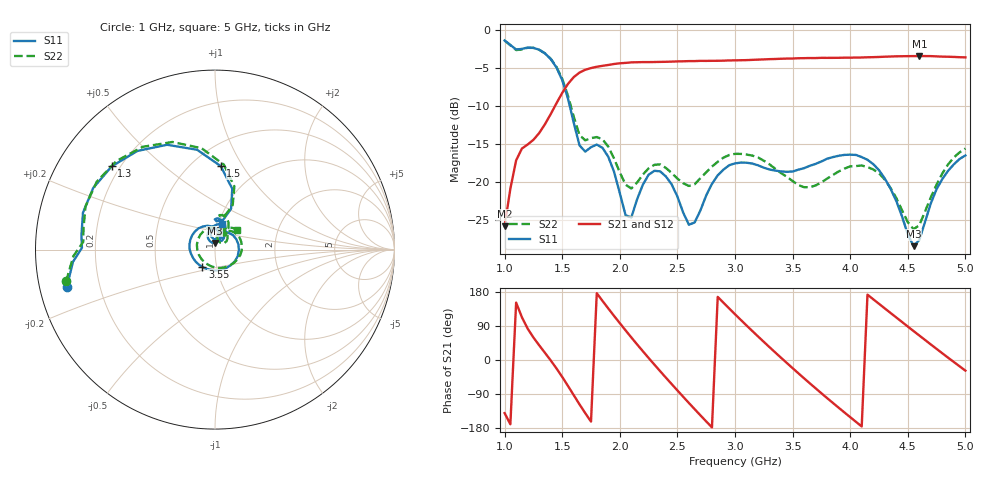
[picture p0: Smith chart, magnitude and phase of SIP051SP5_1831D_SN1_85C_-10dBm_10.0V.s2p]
# GHz  S  dB  R  50
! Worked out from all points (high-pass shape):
!   81 points, 1 GHz to 5 GHz, reference 50 ohm
!   highest |S21| = -3.46 dB at 4.6 GHz (marker M1); lowest = -25.9 dB at 1 GHz (marker M2)
!   |S21| within 3 dB of the highest: 1.587 GHz to end of sweep
!   lowest |S11| = -28.5 dB at 4.55 GHz (marker M3), VSWR 1.08, Z = 49.8 + j3.75 ohm
!   |S11| at or under -10 dB: 1.565 GHz to end of sweep
!   |S22| runs from -26.3 to -1.4 dB; largest |S21 - S12| = 0.0022
!   S11 on the Smith chart (normalised r, x): 1 GHz: 0.08, -0.12; 1.3 GHz: 0.17, +0.34; 1.5 GHz: 0.68, +0.81; 3.55 GHz: 0.85, -0.17; 5 GHz: 1.03, +0.30
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1  -1.41 -165.9  -25.87 -140.1  -25.91 -139.9  -1.43 -167.9
1.1  -2.60 179.3  -17.20 151.5  -17.20 151.5  -2.67 176.6
1.3  -2.62 141.1  -13.60 38.8  -13.58 38.8  -2.64 138.0
1.5  -6.62 86.1  -8.31 -44.6  -8.29 -44.6  -6.45 84.0
1.7  -16.05 86.8  -5.27 -140.2  -5.26 -140.3  -14.55 81.5
1.85  -15.55 76.9  -4.75 155.9  -4.73 155.9  -14.42 71.4
2  -21.51 58.7  -4.42 97.2  -4.40 97.2  -18.77 58.0
2.1  -24.70 95.7  -4.29 59.6  -4.29 59.7  -20.90 75.1
2.2  -20.40 104.5  -4.25 23.2  -4.25 23.2  -19.06 82.4
2.35  -18.64 76.7  -4.23 -29.4  -4.22 -29.3  -17.72 66.5
2.55  -24.07 52.4  -4.15 -96.9  -4.13 -97.0  -20.20 53.7
2.75  -21.82 80.8  -4.10 -162.1  -4.08 -162.1  -18.77 60.2
3  -17.59 26.4  -4.03 120.8  -4.01 120.8  -16.34 26.3
3.3  -18.40 -59.6  -3.87 33.8  -3.86 33.7  -17.72 -33.1
3.55  -18.42 -125.9  -3.75 -35.0  -3.74 -35.1  -20.45 -104.8
3.7  -17.66 -159.7  -3.72 -74.7  -3.71 -74.7  -20.50 -161.7
4.05  -16.48 127.5  -3.66 -163.1  -3.65 -163.2  -17.94 95.9
4.35  -20.92 73.2  -3.52 124.2  -3.53 124.2  -20.81 40.6
4.55  -28.49 91.6  -3.47 76.4  -3.46 76.5  -26.26 54.1
4.6  -27.67 112.3  -3.46 64.6  -3.46 64.5  -25.73 69.7
4.8  -19.64 111.8  -3.54 17.6  -3.52 17.7  -18.91 71.8
5  -16.55 75.6  -3.63 -28.0  -3.63 -28.1  -15.63 42.5
